TYPE ConfigMfcGas :
STRUCT
	Enable:BOOL;
	GasName:STRING;
	DefaultSV:SVINT;
	FlowRegulationFactor:SVINT;
	EnableAlarm:BOOL;
	AlarmRange:SVINT;
	AlarmTime:SVINT;
	WarningRange:SVINT;
	WarningTime:SVINT;
	WriteMode:SVINT;
END_STRUCT
END_TYPE
